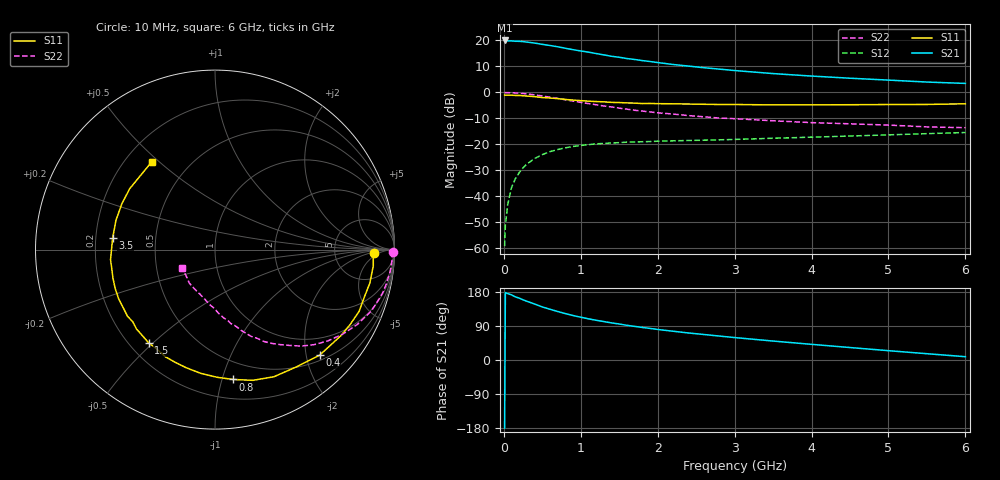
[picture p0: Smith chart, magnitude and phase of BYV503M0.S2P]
! SIEMENS Small Signal Semiconductors
! BFY420
! Si NPN RF SIEGET Grounded Emitter Transistor in MICRO-X
! VCE = 0.5 V  IC = 3 mA
! Common Emitter S-Parameters:  October  1996
# GHz  S  MA  R  50
!  f  S11  S21  S12  S22
! GHz  MAG  ANG  MAG  ANG  MAG  ANG  MAG  ANG
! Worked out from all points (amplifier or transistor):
!   36 points, 10 MHz to 6 GHz, reference 50 ohm
!   highest |S21| = 20.0 dB at 10 MHz (marker M1)
!   |S21| within 3 dB of that: start of sweep to 799.3 MHz
!   unconditionally stable (mu >= 1): 3.449 GHz to end of sweep
!   at 250 MHz: K = 0.08, MSG = 24.3 dB, |S12| = -29.0 dB
!   at 1.4 GHz: K = 0.43, MSG = 16.7 dB, |S12| = -19.5 dB
!   at 6 GHz: K = 1.24, MAG = 6.5 dB, |S12| = -15.4 dB
!   S11 on the Smith chart (normalised r, x): 10 MHz: 16, -3; 400 MHz: 0.61, -2.27; 800 MHz: 0.35, -1.09; 1.5 GHz: 0.28, -0.48; 3.5 GHz: 0.27, +0.05; 6 GHz: 0.31, +0.47
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0.01  0.8855 -1.3  9.973 -179.7  0.0011 96.2  0.9899 -0.7
0.02  0.8825 -2.5  9.938 178.0  0.0028 85.9  0.9878 -1.4
0.05  0.8866 -5.9  9.791 175.2  0.0069 86.1  0.9879 -3.6
0.1  0.8826 -12.2  9.768 171.8  0.0148 83.9  0.9833 -7.3
0.15  0.8733 -17.4  9.624 166.6  0.0219 79.0  0.9746 -11.0
0.2  0.8735 -23.2  9.598 163.2  0.0286 76.8  0.9646 -14.5
0.25  0.8608 -29.0  9.478 158.8  0.0354 73.1  0.949 -18.0
0.4  0.8282 -45.2  8.89 147.8  0.0535 63.9  0.8963 -27.7
0.5  0.7955 -55.2  8.384 140.0  0.0635 58.7  0.8528 -33.6
0.6  0.7808 -65.1  7.975 133.9  0.0725 54.0  0.8085 -39.0
0.8  0.7307 -82.0  7.057 122.4  0.0858 45.5  0.7211 -48.2
0.9  0.7113 -89.1  6.631 117.3  0.091 42.3  0.6799 -51.8
1.1  0.6776 -103.6  5.943 108.7  0.0986 36.5  0.6083 -59.1
1.3  0.658 -114.9  5.265 101.4  0.1043 31.9  0.5471 -64.6
1.5  0.6375 -125.5  4.735 95.0  0.1079 28.3  0.4976 -69.6
1.8  0.6095 -138.7  4.088 85.9  0.1124 24.5  0.4365 -75.5
2.2  0.6028 -152.9  3.439 75.9  0.1171 20.5  0.3831 -82.8
2.8  0.5846 -170.0  2.804 63.2  0.1223 17.3  0.3208 -92.1
3.5  0.5739 173.7  2.299 50.0  0.1311 14.7  0.2842 -101.1
4.5  0.5784 153.8  1.872 32.9  0.1446 10.6  0.2485 -116.6
5.5  0.5862 134.4  1.58 16.6  0.1607 6.0  0.2168 -138.4
6  0.6031 125.6  1.488 8.7  0.169 3.7  0.2091 -151.3
